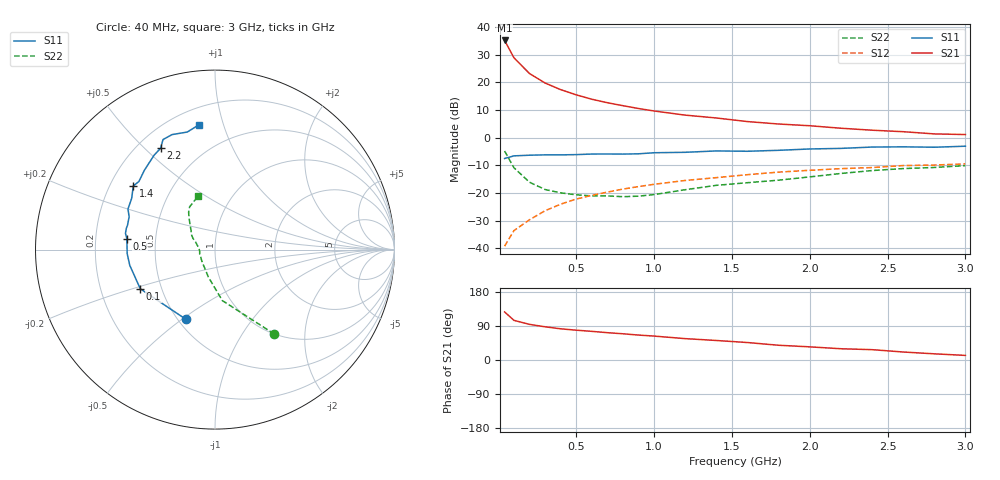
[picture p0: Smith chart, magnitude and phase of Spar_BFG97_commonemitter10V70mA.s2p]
! Filename:  BFG97H.S2P  Version:  2.0
! NXP part #: BFG97  Date: Jul 1990
! Bias condition: Vce=10V, Ic=70mA
#  MHz  S  MA  R  50
! Freq  S11  S21  S12  S22  !GUM [dB]
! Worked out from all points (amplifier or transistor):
!   21 points, 40 MHz to 3 GHz, reference 50 ohm
!   highest |S21| = 35.1 dB at 40 MHz (marker M1)
!   |S21| within 3 dB of that: start of sweep to 68.77 MHz
!   unconditionally stable (mu >= 1): 195.3 MHz to 2.488 GHz; 2.623 GHz to 2.952 GHz
!   at 300 MHz: K = 1.04, MAG = 21.8 dB, |S12| = -26.4 dB
!   at 1 GHz: K = 1.08, MAG = 11.6 dB, |S12| = -16.8 dB
!   at 3 GHz: K = 0.99, MSG = 5.3 dB, |S12| = -9.5 dB
!   S11 on the Smith chart (normalised r, x): 40 MHz: 0.55, -0.52; 100 MHz: 0.38, -0.21; 500 MHz: 0.34, +0.05; 1.4 GHz: 0.30, +0.32; 2.2 GHz: 0.29, +0.56; 3 GHz: 0.30, +0.84
40  0.421 -112.5  57.02 126.8  0.011 60.6  0.575 -54.9
100  0.47 -152.3  27.74 104.6  0.021 61.0  0.287 -81.8
200  0.483 -169.6  14.4 94.0  0.033 69.8  0.157 -103.7
300  0.49 -177.5  9.723 87.6  0.048 71.9  0.116 -120.3
400  0.49 178.8  7.379 82.3  0.063 71.2  0.101 -134.4
500  0.495 172.9  5.943 78.7  0.078 71.6  0.093 -145.7
600  0.507 169.7  4.95 75.6  0.091 70.7  0.089 -154.2
700  0.508 166.5  4.283 72.1  0.104 70.2  0.089 -163.4
800  0.506 164.4  3.784 69.2  0.118 68.3  0.086 -172.8
900  0.512 159.1  3.367 65.8  0.131 67.8  0.088 178.6
1000  0.535 155.0  3.038 63.1  0.144 65.7  0.094 171.6
1200  0.545 148.4  2.556 56.4  0.169 63.7  0.115 159.1
1400  0.577 142.1  2.27 51.5  0.19 60.2  0.138 153.0
1600  0.569 138.2  1.955 46.1  0.215 58.8  0.154 147.9
1800  0.592 131.6  1.767 38.9  0.239 54.3  0.171 141.3
2000  0.626 122.8  1.644 34.7  0.258 51.7  0.196 135.2
2200  0.641 118.2  1.483 29.7  0.276 49.4  0.226 129.6
2400  0.678 115.3  1.366 27.3  0.289 48.1  0.255 125.2
2600  0.684 110.5  1.284 21.1  0.314 44.0  0.277 120.7
2800  0.673 103.3  1.171 16.3  0.321 39.7  0.29 114.8
3000  0.702 97.1  1.14 12.1  0.336 38.0  0.313 107.2
